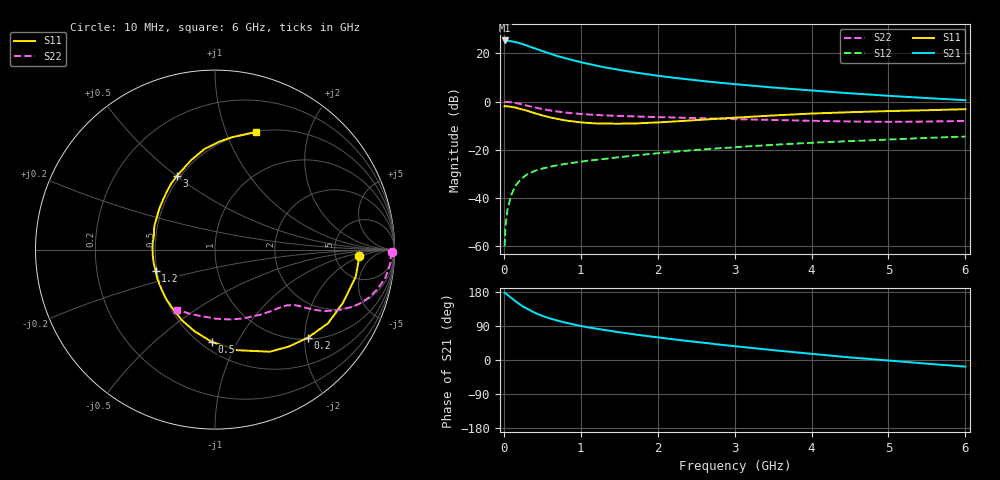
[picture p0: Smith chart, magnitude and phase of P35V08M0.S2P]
! SIEMENS Small Signal Semiconductors
! BFP181
! Si NPN RF Bipolar Junction Transistor in SOT143
! VCE = 5 V  IC = 8 mA
! Common Emitter S-Parameters:  March  1996
# GHz  S  MA  R  50
!  f  S11  S21  S12  S22
! GHz  MAG  ANG  MAG  ANG  MAG  ANG  MAG  ANG
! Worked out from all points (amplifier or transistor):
!   36 points, 10 MHz to 6 GHz, reference 50 ohm
!   highest |S21| = 25.3 dB at 10 MHz (marker M1)
!   |S21| within 3 dB of that: start of sweep to 377.9 MHz
!   unconditionally stable (mu >= 1): 1.393 GHz to end of sweep
!   at 250 MHz: K = 0.29, MSG = 27.6 dB, |S12| = -31.5 dB
!   at 1.4 GHz: K = 1.00, MAG = 18.3 dB, |S12| = -23.5 dB
!   at 6 GHz: K = 1.02, MAG = 6.7 dB, |S12| = -14.5 dB
!   S11 on the Smith chart (normalised r, x): 10 MHz: 8.72, -1.63; 200 MHz: 1.03, -2.07; 500 MHz: 0.57, -0.79; 1.2 GHz: 0.49, -0.13; 3 GHz: 0.48, +0.50; 6 GHz: 0.51, +1.28
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0.01  0.8005 -2.4  18.5 177.8  0.001 88.8  0.9853 -0.8
0.02  0.8029 -4.5  18.33 176.7  0.0025 92.4  0.9808 -1.8
0.05  0.7981 -11.0  18.3 171.4  0.0061 86.4  0.9786 -4.8
0.1  0.7721 -22.6  17.73 163.3  0.0119 76.3  0.9624 -9.4
0.15  0.7519 -33.1  17.09 155.3  0.0179 72.4  0.9326 -13.5
0.2  0.7126 -43.6  16.4 147.9  0.0223 69.1  0.899 -17.3
0.25  0.6788 -52.7  15.38 141.1  0.0266 64.5  0.8597 -20.5
0.3  0.646 -61.7  14.48 135.8  0.0305 61.4  0.824 -22.9
0.4  0.5743 -77.5  12.73 124.9  0.0364 56.2  0.7565 -26.7
0.5  0.5152 -91.9  11.13 116.4  0.0408 52.3  0.6991 -29.3
0.6  0.4692 -104.0  9.902 109.6  0.0444 50.2  0.6536 -31.0
0.7  0.4351 -115.0  8.735 103.9  0.0478 48.5  0.6194 -32.1
0.8  0.405 -125.3  7.929 98.7  0.0509 47.6  0.593 -32.9
1.1  0.3602 -152.9  6.05 86.0  0.0596 46.2  0.5389 -35.0
1.2  0.3518 -160.2  5.574 82.8  0.0618 46.0  0.5278 -35.9
1.7  0.3493 167.2  4.028 67.6  0.0761 45.1  0.4913 -40.6
2.2  0.3847 143.8  3.129 54.7  0.0905 43.1  0.4671 -46.7
3  0.4621 117.4  2.299 36.5  0.1128 38.7  0.4313 -58.7
3.5  0.5144 105.2  1.955 26.0  0.1267 35.5  0.415 -67.7
4.5  0.6009 87.9  1.484 6.8  0.1511 28.1  0.3857 -88.7
5.5  0.6604 75.8  1.18 -9.7  0.1761 21.5  0.3844 -111.0
6  0.6947 70.7  1.067 -17.5  0.1879 17.5  0.3957 -122.4
